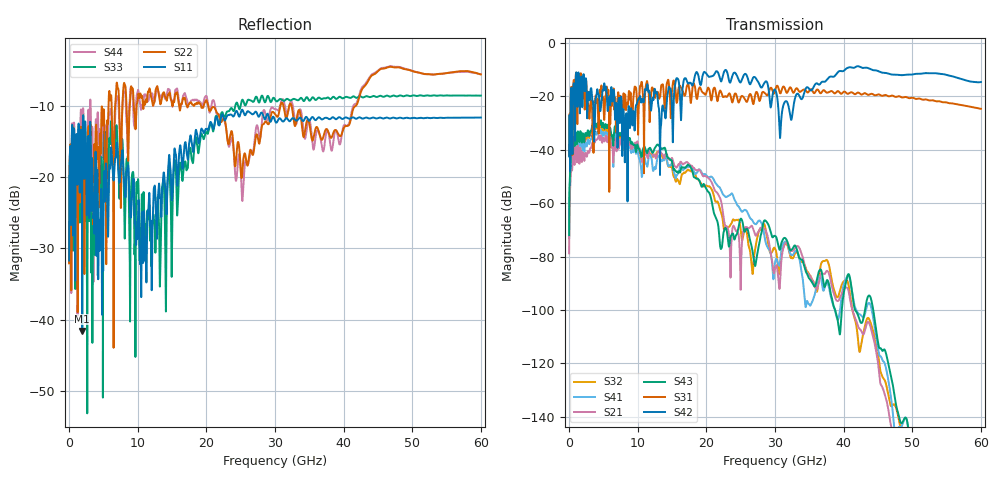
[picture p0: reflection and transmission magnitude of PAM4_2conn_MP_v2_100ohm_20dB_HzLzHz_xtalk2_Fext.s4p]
! Info: Touchstone file created by Circ.  Input file=FAB50GbE_2conn_Midplane_Examax_Topo2_v2_100ohm_20dB_HzLzHz.circ
# Hz S RI R 50
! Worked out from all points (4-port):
!   6000 points, 10 MHz to 60 GHz, reference 50 ohm
!   strongest paths, dB at 10 MHz, 15.01 GHz, 30.01 GHz, 45.01 GHz, 60 GHz:
!     S42: -42.5, -25.2, -17.5, -10.5, -14.7
!     S31: -42.0, -17.8, -17.9, -19.3, -24.7
!     S43: -71.9, -44.6, -72.3, -112.1, -157.9
!     S21: -78.9, -43.1, -84.5, -119.8, -163.6
!     S41: -72.5, -44.8, -82.4, -114.5, -167.8
!     S32: -73.1, -46.7, -77.0, -116.2, -161.0
!   lowest |S11| = -41.6 dB at 1.9 GHz (marker M1), VSWR 1.02, Z = 49.6 - j0.703 ohm
!   |S11| at or under -10 dB: start of sweep to end of sweep
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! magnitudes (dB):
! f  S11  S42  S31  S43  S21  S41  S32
! 10 MHz  -31.7  -42.5  -42.0  -71.9  -78.9  -72.5  -73.1
! 460 MHz  -12.6  -28.3  -27.4  -40.9  -47.3  -44.6  -42.4
! 1.9 GHz  -41.6  -19.9  -21.0  -36.5  -43.7  -39.5  -37.9
! 8.3 GHz  -21.3  -27.3  -25.1  -36.0  -38.7  -39.3  -37.1
! 27.1 GHz  -10.8  -12.9  -19.7  -83.6  -71.7  -67.8  -77.6
! 30.8 GHz  -11.8  -33.6  -18.9  -76.6  -86.5  -80.9  -81.9
! 60 GHz  -11.6  -14.7  -24.7  -157.9  -163.6  -167.8  -161.0
